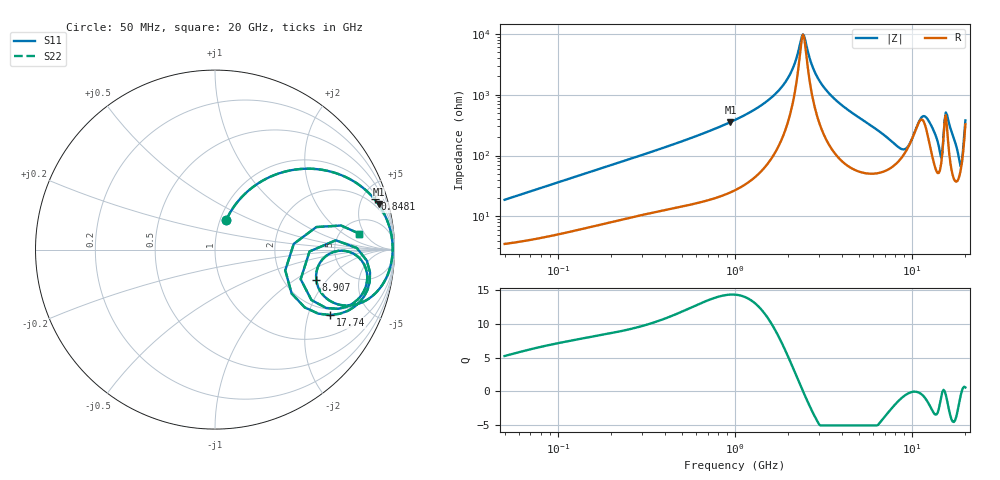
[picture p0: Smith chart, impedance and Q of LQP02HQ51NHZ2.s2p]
!Murata Part Number: LQP02HQ51NHZ2
!These Parameters are Measured in Series Mode Connection
!  o--[Z]--o
!Port1  Port2
!  o-------o
!Freq. Start=50[MHz] Stop=20[GHz], 401[Steps]
# Hz S RI R 50
!Freq.(Hz) S11(Real) S11(Imag) S21(Real) S21(Imag) S12(Real) S12(Imag) S22(Real) S22(Imag)
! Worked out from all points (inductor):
!   401 points, 50 MHz to 20 GHz, reference 50 ohm
!   read as one part in series: L = 58.1 nH near 51.52 MHz
!   highest Q = 14.3 at 941.8 MHz (marker M1), where L = 59.6 nH
!   self-resonance near 2.42 GHz
!   S11 on the Smith chart (normalised r, x): 50 MHz: 1.07, +0.37; 848.1 MHz: 1.44, +6.17; 8.907 GHz: 3.00, -1.53; 17.74 GHz: 1.74, -2.79; 20 GHz: 7.49, +3.84
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5e7  0.0636 0.1664  0.9364 -0.1664  0.9364 -0.1664  0.0636 0.1664
1.364002e8  0.2188 0.3542  0.7812 -0.3542  0.7812 -0.3542  0.2188 0.3542
3.721004e8  0.6055 0.4431  0.3945 -0.4431  0.3945 -0.4431  0.6055 0.4431
8.480927e8  0.8892 0.2804  0.1108 -0.2804  0.1108 -0.2804  0.8892 0.2804
9.418449e8  0.911 0.2519  0.089 -0.2519  0.089 -0.2519  0.911 0.2519
1e9  0.922 0.2354  0.078 -0.2354  0.078 -0.2354  0.922 0.2354
1.820564e9  0.9841 0.0744  0.0159 -0.0744  0.0159 -0.0744  0.9841 0.0744
2.114743e9  0.9888 0.0355  0.0112 -0.0355  0.0112 -0.0355  0.9888 0.0355
2.419936e9  0.9899 0.000501  0.0101 -0.000501  0.0101 -0.000501  0.9899 0.000501
2.728004e9  0.9882 -0.0311  0.0118 0.0311  0.0118 0.0311  0.9882 -0.0311
3.736399e9  0.9699 -0.1186  0.0301 0.1186  0.0301 0.1186  0.9699 -0.1186
7.442007e9  0.7138 -0.3107  0.2862 0.3107  0.2862 0.3107  0.7138 -0.3107
8.907419e9  0.564 -0.1674  0.436 0.1674  0.436 0.1674  0.564 -0.1674
1.019291e10  0.6833 -0.0074  0.3167 0.0074  0.3167 0.0074  0.6833 -0.0074
1.149051e10  0.8284 -0.0785  0.1716 0.0785  0.1716 0.0785  0.8284 -0.0785
1.314879e10  0.8135 -0.2575  0.1865 0.2575  0.1865 0.2575  0.8135 -0.2575
1.438523e10  0.5374 -0.281  0.4626 0.281  0.4626 0.281  0.5374 -0.281
1.504638e10  0.673 0.0518  0.327 -0.0518  0.327 -0.0518  0.673 0.0518
1.573793e10  0.8637 -0.1267  0.1363 0.1267  0.1363 0.1267  0.8637 -0.1267
1.774144e10  0.6417 -0.3647  0.3583 0.3647  0.3583 0.3647  0.6417 -0.3647
1.88369e10  0.3915 -0.1156  0.6085 0.1156  0.6085 0.1156  0.3915 -0.1156
2e10  0.8045 0.0884  0.1955 -0.0884  0.1955 -0.0884  0.8045 0.0884
